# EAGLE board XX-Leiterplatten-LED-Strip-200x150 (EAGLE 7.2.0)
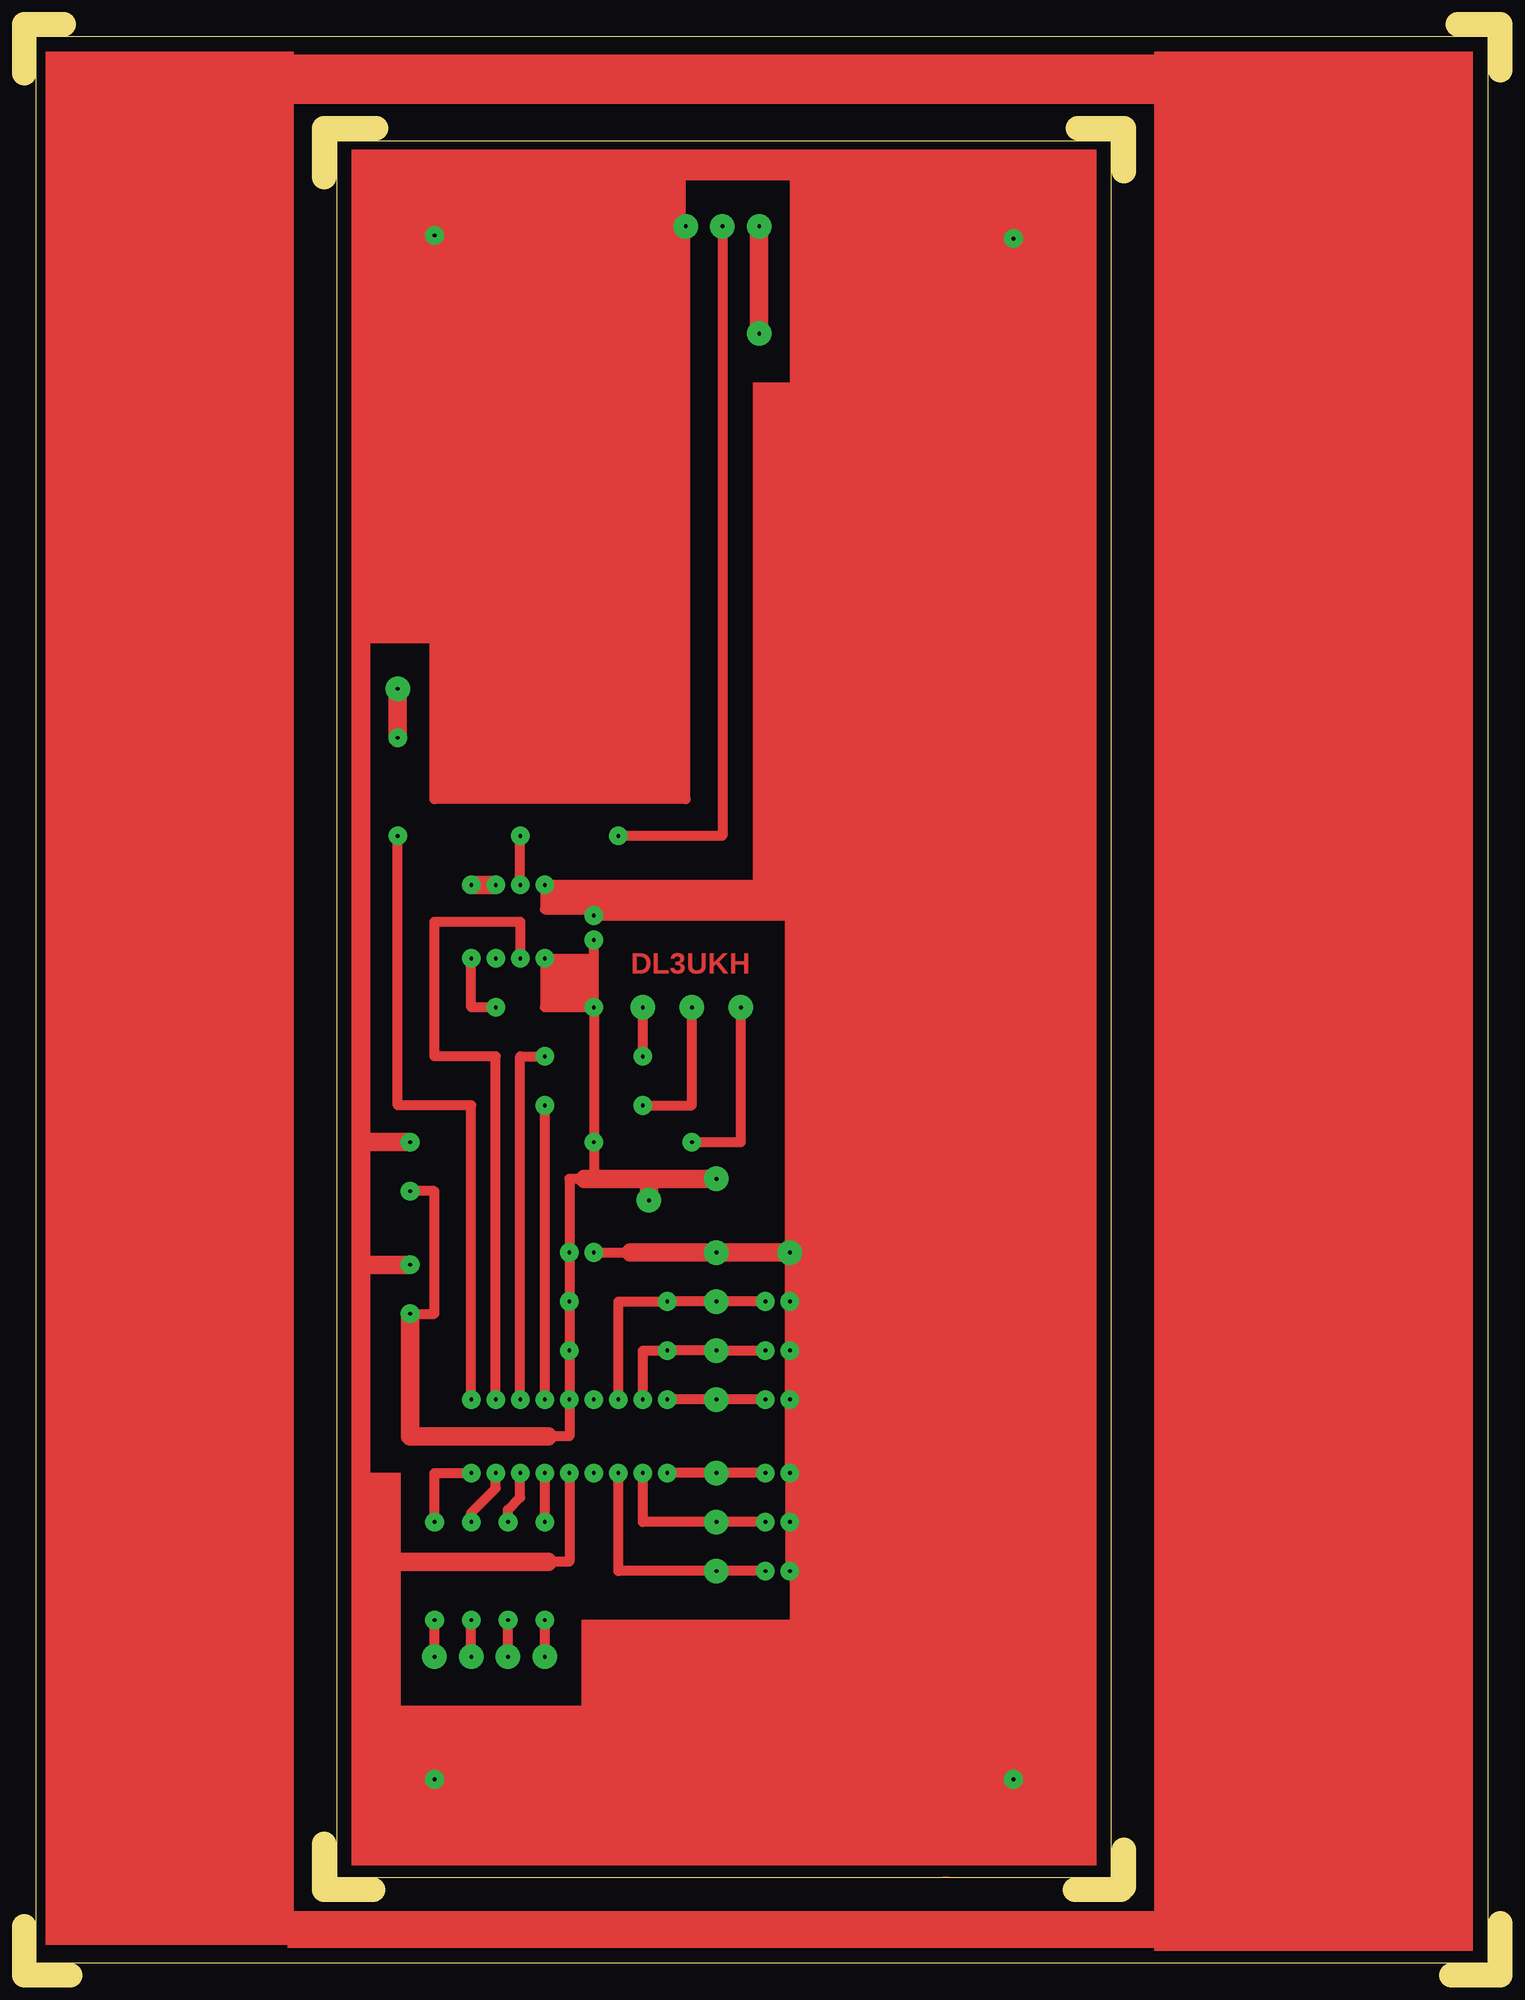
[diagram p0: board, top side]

Size 153.03 x 202.25 mm. Coordinates in mm from the lower left corner, seen from the top.
Outline: 153.03,5.4 153.03,0.32
Outline: 153.03,0 147.96,0
Outline: 153.03,197.49 153.03,202.25 148.59,202.25
Outline: 0,5.08 0,0 4.76,0
Outline: 4.13,202.25 0,202.25
Outline: 0,197.17 0,201.93
Outline: 36.51,191.45 31.43,191.45
Outline: 31.11,191.45 31.11,186.37
Outline: 109.22,191.45 113.98,191.45 113.98,187.01
Outline: 36.2,8.89 31.11,8.89 31.11,13.65
Outline: 113.98,13.02 113.98,9.21
Outline: 108.9,8.89 113.66,8.89
Outline: 151.77,1.27 151.77,200.98 1.27,200.98 1.27,1.27 151.77,1.27
Outline: 32.38,190.18 112.71,190.18 112.71,10.16 32.38,10.16 32.38,190.18
Copper layers (1*16): Top 0.035mm / dielectric 1.5mm / Bottom 0.035mm
Design rules "default": minimum track width 10mil, minimum drill 24mil, track to track 8mil, track to pad 8mil, pad to pad 8mil, via to via 8mil, smd to smd 8mil, copper to edge 40mil, drill to drill 8mil, minimum pad ring 10mil, minimum via ring 8mil, stop-mask expansion 4mil, vias tented up to drill 0mil, thermal gap 10mil

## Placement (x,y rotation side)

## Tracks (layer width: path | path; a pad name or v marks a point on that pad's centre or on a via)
S$1
  Top 1.016: 72.39,181.61 72.39,118.11 61.28,118.11
S$2  (via drill 0.4 pad 1.93)
  Top 1.016: v53.98,113.03 53.98,110.49 59.37,110.49
S$3  (via drill 0.4 pad 1.93, 0.4 pad 2.54)
  Top 1.016: 59.05,82.55 v59.05,86.36 v59.05,100.33 53.98,100.33 v53.98,105.41 59.05,105.41 | 59.05,82.55 58.1,82.55 56.52,82.55 v56.52,74.93 v56.52,69.85 v56.52,64.77 v56.52,59.69 56.52,55.88 54.29,55.88 | v40.01,68.58 42.55,68.58 42.55,81.28 v40.01,81.28 | v71.75,82.55 64.77,82.55 59.05,82.55 | 59.05,100.65 59.05,105.41 | 59.05,105.41 59.05,107.63
  Top 1.93: v64.77,80.33 64.77,82.55 | v40.01,68.58 40.01,55.88 54.29,55.88 | v71.75,82.55 58.1,82.55
S$4  (via drill 0.4 pad 1.93)
  other vias: 102.55,180.02
S$6
  Top 0: 95.88,10.16 95.25,10.16
S$10  (via drill 0.4 pad 1.93)
  other vias: 42.55,180.34
S$12  (via drill 0.4 pad 1.93)
  other vias: 42.55,20.32
S$13  (via drill 0.4 pad 1.93)
  Top 1.016: v53.98,59.69 v53.98,90.17
S$14  (via drill 0.4 pad 1.93)
  other vias: 51.44,118.11
S$15  (via drill 0.4 pad 1.93)
  Top 1.016: v53.98,46.99 v53.98,52.07
S$19  (via drill 0.4 pad 1.93)
  other vias: 59.05,52.07
S$22  (via drill 0.4 pad 1.93)
  other vias: 102.55,20.32
S$23  (via drill 0.4 pad 1.93)
  other vias: 61.6,118.11
S$29  (via drill 0.4 pad 1.93)
  other vias: 59.05,107.31
S$30  (via drill 0.4 pad 2.54)
  Top 1.93: v76.2,181.29 v76.2,170.18
S$32  (via drill 0.4 pad 1.93, 0.4 pad 2.54)
  Top 1.016: v69.21,86.36 74.3,86.36 v74.3,100.33
S$34  (via drill 0.4 pad 1.93)
  Top 1.016: v46.36,59.69 46.36,90.17 38.74,90.17 v38.74,118.11
S$35  (via drill 0.4 pad 1.93)
  Top 1.016: v50.17,46.99 50.17,48.26 51.44,49.53 v51.44,52.07
S$36  (via drill 0.4 pad 2.54)
  other vias: 72.39,181.29
S$37  (via drill 0.4 pad 1.93, 0.4 pad 2.54)
  Top 1.016: v56.52,52.07 56.52,42.86 54.29,42.86 | 35.88,42.86 34.93,42.86 34.93,73.66 34.93,86.36 34.93,146.05 42.55,146.05 | 42.55,146.05 42.55,121.92 68.58,121.92 | 42.55,146.05 68.58,121.92 | 68.58,121.92 v68.58,181.29
  Top 1.93: v40.01,73.66 34.93,73.66 | v40.01,86.36 34.93,86.36 | 35.88,42.86 54.29,42.86
S$39  (via drill 0.4 pad 1.93)
  Top 1.016: v48.9,59.69 48.9,95.25 42.55,95.25 42.55,109.22 51.44,109.22 v51.44,105.41
S$40  (via drill 0.4 pad 1.93)
  other vias: 59.05,59.69
S$43  (via drill 0.4 pad 1.93, 0.4 pad 2.54)
  Top 1.016: 53.98,33.97 v53.98,33.02 v53.98,36.83
S$44  (via drill 0.4 pad 1.93)
  other vias: 66.67,59.69
S$45  (via drill 0.4 pad 1.93)
  Top 1.93: v48.9,113.03 v46.36,113.03
S$46  (via drill 0.4 pad 1.93)
  Top 1.016: v46.36,46.99 46.36,47.94 48.9,50.48 v48.9,52.07
S$47  (via drill 0.4 pad 1.93)
  other vias: 51.44,113.03
S$48  (via drill 0.4 pad 1.93)
  Top 1.016: v42.55,46.99 42.55,52.07 v46.36,52.07
S$49  (via drill 0.4 pad 1.93)
  other vias: 48.9,105.41
S$50
  Top 1.016: 51.44,113.35 51.44,118.11
S$52  (via drill 0.4 pad 1.93, 0.4 pad 2.54)
  Top 1.016: v50.17,33.02 v50.17,36.83
S$53  (via drill 0.4 pad 1.93, 0.4 pad 2.54)
  Top 1.016: v64.14,90.17 69.21,90.17 v69.21,100.33
S$54  (via drill 0.4 pad 1.93, 0.4 pad 2.54)
  Top 1.016: v64.14,95.25 v64.14,100.33
S$56  (via drill 0.4 pad 1.93)
  Top 1.016: v48.9,100.33 46.36,100.33 v46.36,105.41
S$58  (via drill 0.4 pad 1.93, 0.4 pad 2.54)
  Top 1.93: v38.74,128.27 v38.74,133.35
S$59  (via drill 0.4 pad 1.93, 0.4 pad 2.54)
  Top 1.016: v46.36,33.02 v46.36,36.83
S$63  (via drill 0.4 pad 1.93, 0.4 pad 2.54)
  Top 1.016: v42.55,33.02 v42.55,36.83
S$68  (via drill 0.4 pad 1.93, 0.4 pad 2.54)
  Top 1.016: v64.14,59.69 64.14,64.77 v66.67,64.77 v71.75,64.77 v76.83,64.77
S$70  (via drill 0.4 pad 1.93)
  Top 1.016: v51.44,59.69 51.44,95.25 v53.98,95.25
S$71  (via drill 0.4 pad 1.93, 0.4 pad 2.54)
  Top 1.016: v61.6,59.69 61.6,69.85 v66.67,69.85 v71.75,69.85 v76.83,69.85
S$72  (via drill 0.4 pad 2.54)
  other vias: 71.75,59.69
S$74  (via drill 0.4 pad 1.93)
  Top 1.016: v76.83,59.69 66.36,59.69
S$76  (via drill 0.4 pad 2.54)
  other vias: 71.75,52.07
S$77  (via drill 0.4 pad 2.54)
  other vias: 71.75,46.99
S$78  (via drill 0.4 pad 2.54)
  other vias: 71.75,41.91
S$80  (via drill 0.4 pad 1.93)
  Top 1.016: v76.83,52.07 v66.67,52.07
S$82  (via drill 0.4 pad 1.93, 0.4 pad 2.54)
  Top 1.016: v59.05,74.93 62.87,74.93 v71.75,74.93 v79.38,74.93 | v79.38,74.93 79.38,113.03 59.05,113.03 | 59.05,113.03 v59.05,109.85 80.01,109.85 | 59.05,113.03 53.66,113.03 | v79.38,74.93 v79.38,69.85 v79.38,64.77 v79.38,59.69 v79.38,52.07 v79.38,41.91
  Top 1.93: v79.38,74.93 62.87,74.93
S$83  (via drill 0.4 pad 1.93)
  Top 1.016: v76.83,46.99 64.14,46.99 v64.14,52.07
S$84  (via drill 0.4 pad 1.93)
  other vias: 79.38,46.99
S$85  (via drill 0.4 pad 1.93)
  Top 1.016: v76.83,41.91 61.6,41.91 v61.6,52.07
(copper drawn outside any net)
  shapes: Top area x19

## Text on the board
Top: DL3UKH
